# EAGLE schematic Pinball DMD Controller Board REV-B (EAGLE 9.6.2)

## Sheet 1 of 6: Clock / Sync
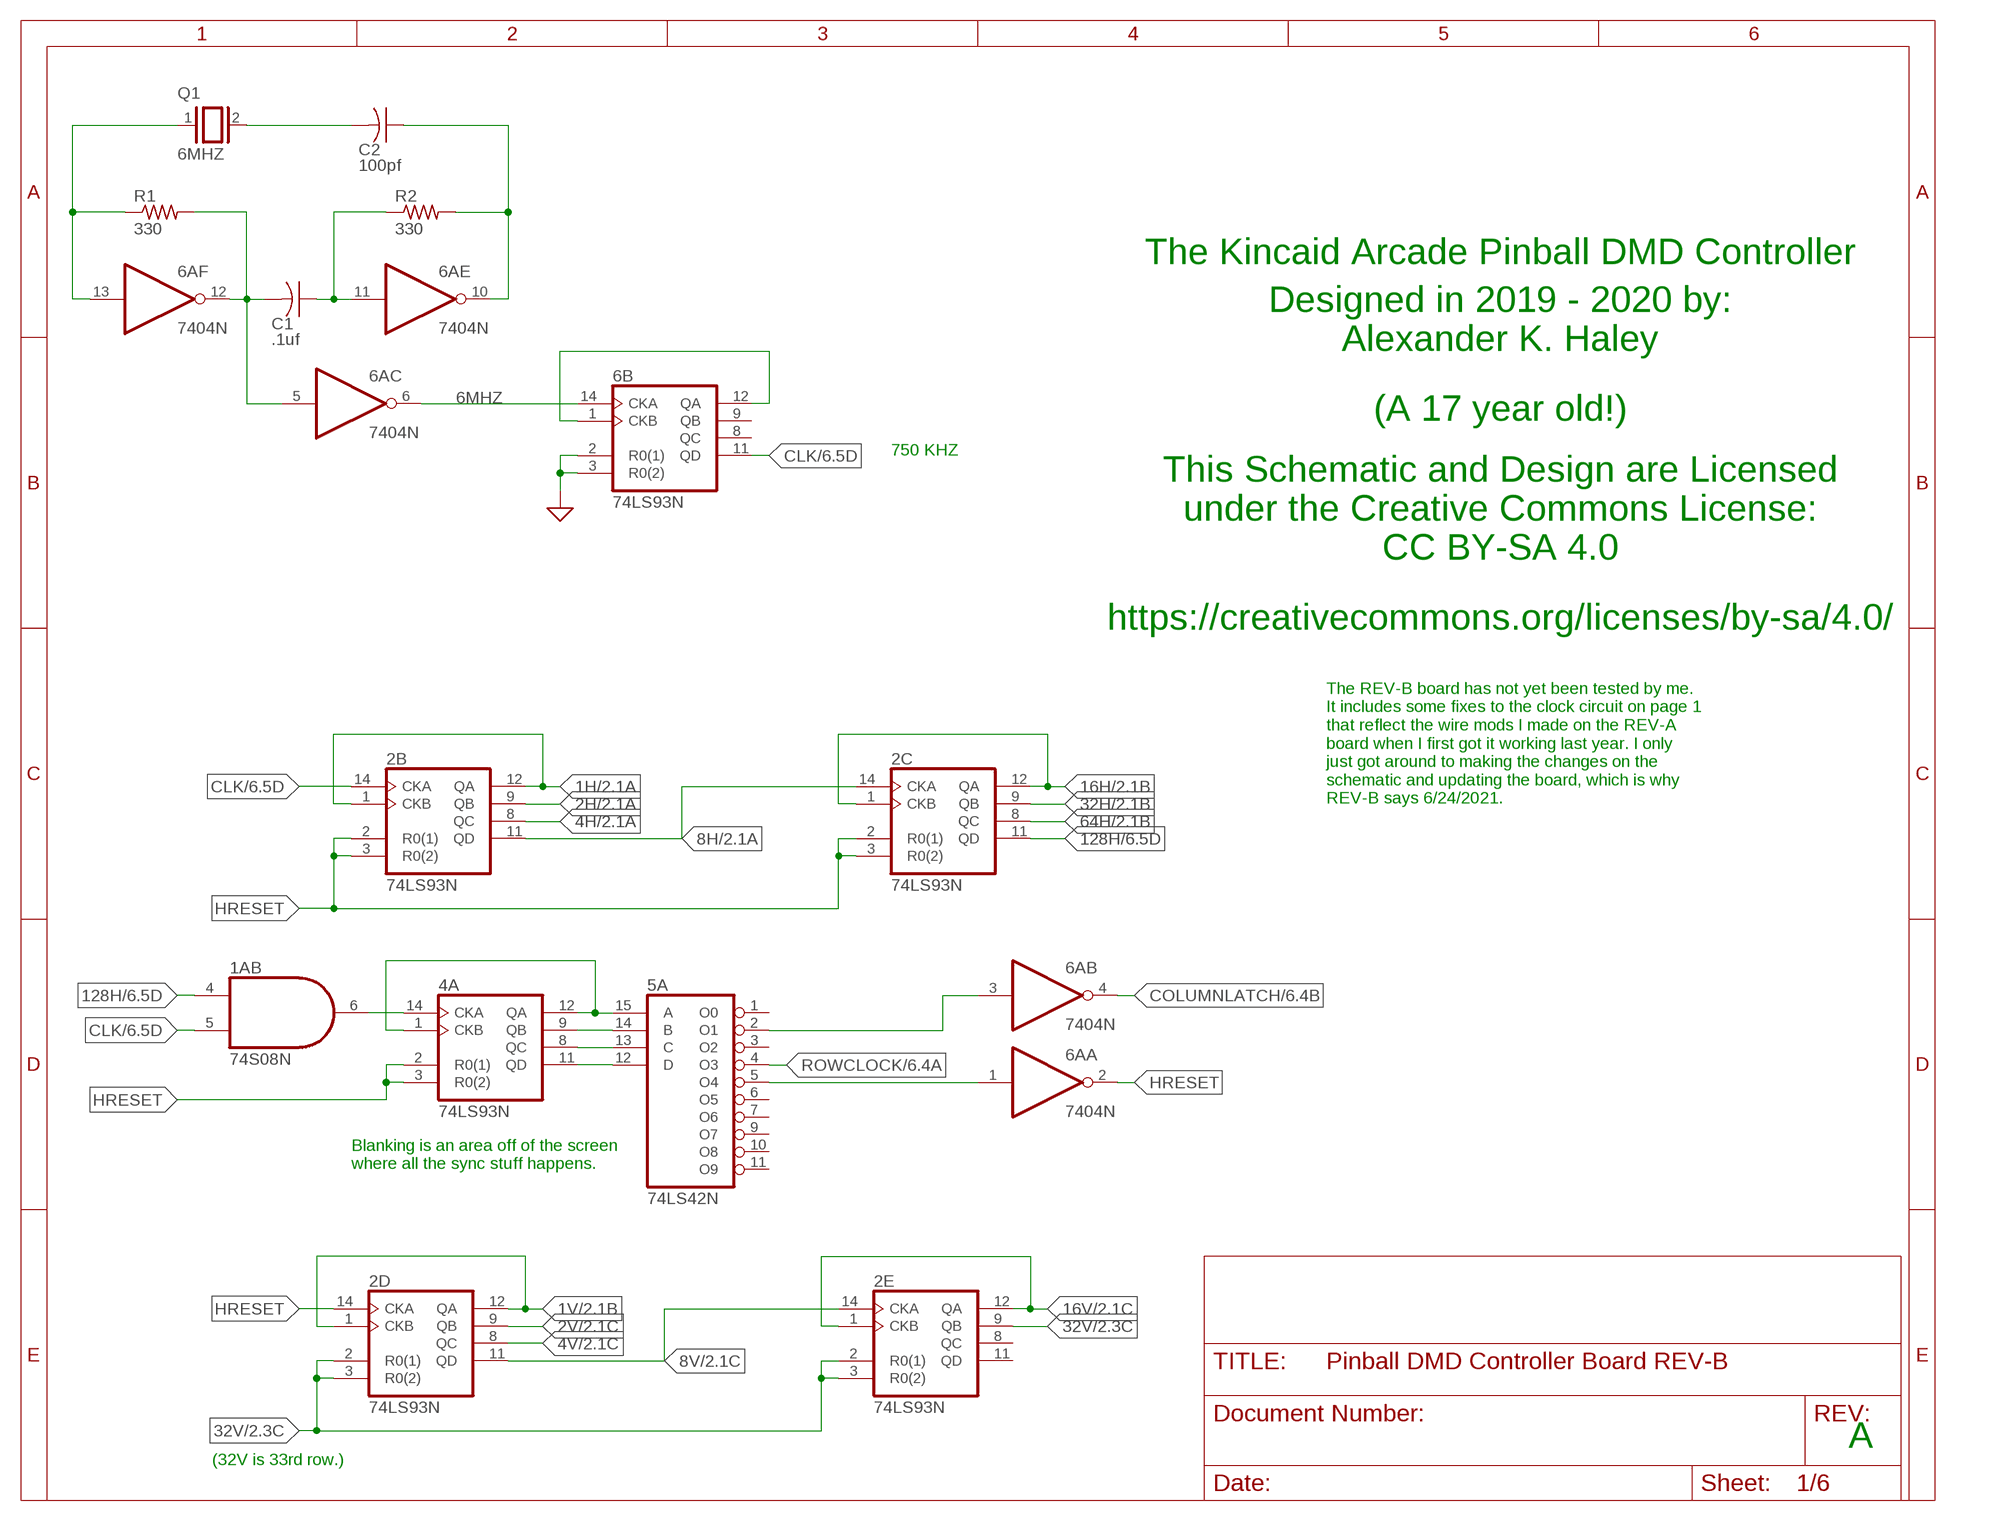
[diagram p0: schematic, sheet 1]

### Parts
1A  74S08N  [DIL14]
2B  74LS93N  [DIL14]
2C  74LS93N  [DIL14]
2D  74LS93N  [DIL14]
2E  74LS93N  [DIL14]
4A  74LS93N  [DIL14]
5A  74LS42N  [DIL16]
6A  7404N  [DIL14]
6B  74LS93N  [DIL14]
C1  .1uf  C-US050-025X075  [C050-025X075]
C2  100pf  C-US050-025X075  [C050-025X075]
Q1  6MHZ  XTAL/S  [QS]
R1  330  R-US_0204/7  [0204/7]
R2  330  R-US_0204/7  [0204/7]

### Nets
1H: 2B.1(CKB) 2B.12(QA) ; also sheet 2,3
1V: 2D.1(CKB) 2D.12(QA) ; also sheet 2,3,6
2H: 2B.9(QB) ; also sheet 2,3
2V: 2D.9(QB) ; also sheet 2,3,6
4H: 2B.8(QC) ; also sheet 2,3
4V: 2D.8(QC) ; also sheet 2,3,6
6MHZ: 6A.6(C:O) 6B.14(CKA) ; also sheet 4
8H: 2B.11(QD) 2C.14(CKA) ; also sheet 2,3
8V: 2D.11(QD) 2E.14(CKA) ; also sheet 2,3,6
16H: 2C.1(CKB) 2C.12(QA) ; also sheet 2,3
16V: 2E.1(CKB) 2E.12(QA) ; also sheet 2,3,6
32H: 2C.9(QB) ; also sheet 2,3
32V: 2D.2(R0(1)) 2D.3(R0(2)) 2E.2(R0(1)) 2E.3(R0(2)) 2E.9(QB) ; also sheet 2
64H: 2C.8(QC) ; also sheet 2,3
128H: 1A.4(B:I0) 2C.11(QD) ; also sheet 6
CLK: 1A.5(B:I1) 2B.14(CKA) 6B.11(QD) ; also sheet 6
COLUMNLATCH: 6A.4(B:O) ; also sheet 6
GND: 6B.2(R0(1)) 6B.3(R0(2)) ; supply symbol labelled SUP ; also sheet 2,3,4,5,6
HRESET: 2B.2(R0(1)) 2B.3(R0(2)) 2C.2(R0(1)) 2C.3(R0(2)) 2D.14(CKA) 4A.2(R0(1)) 4A.3(R0(2)) 6A.2(A:O)
N$1: 6A.13(F:I) Q1.1 R1.1
N$2: 6A.5(C:I) 6A.12(F:O) C1.2 R1.2
N$3: 6A.11(E:I) C1.1 R2.1
N$4: C2.2 Q1.2
N$5: 6A.10(E:O) C2.1 R2.2
N$7: 6B.1(CKB) 6B.12(QA)
N$14: 1A.6(B:O) 4A.14(CKA)
N$15: 4A.1(CKB) 4A.12(QA) 5A.15(A)
N$17: 4A.9(QB) 5A.14(B)
N$18: 4A.8(QC) 5A.13(C)
N$19: 4A.11(QD) 5A.12(D)
N$20: 5A.5(O4) 6A.1(A:I)
N$21: 5A.2(O1) 6A.3(B:I)
ROWCLOCK: 5A.4(O3) ; also sheet 6
Unconnected: 2E.8(QC) 2E.11(QD) 5A.1(O0) 5A.3(O2) 5A.6(O5) 5A.7(O6) 5A.9(O7) 5A.10(O8) 5A.11(O9) 6B.8(QC) 6B.9(QB)

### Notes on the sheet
- The Kincaid Arcade Pinball DMD Controller
- Designed in 2019 - 2020 by:
  Alexander K. Haley
- (A 17 year old!)
- 750 KHZ
- This Schematic and Design are Licensed
  under the Creative Commons License:
  CC BY-SA 4.0
- https://creativecommons.org/licenses/by-sa/4.0/
- The REV-B board has not yet been tested by me.
  It includes some fixes to the clock circuit on page 1
  that reflect the wire mods I made on the REV-A
  board when I first got it working last year. I only
  just got around to making the changes on the
  schematic and updating the board, which is why
  REV-B says 6/24/2021.
- Blanking is an area off of the screen
  where all the sync stuff happens.
- A
- (32V is 33rd row.)

## Sheet 2 of 6: Memory A
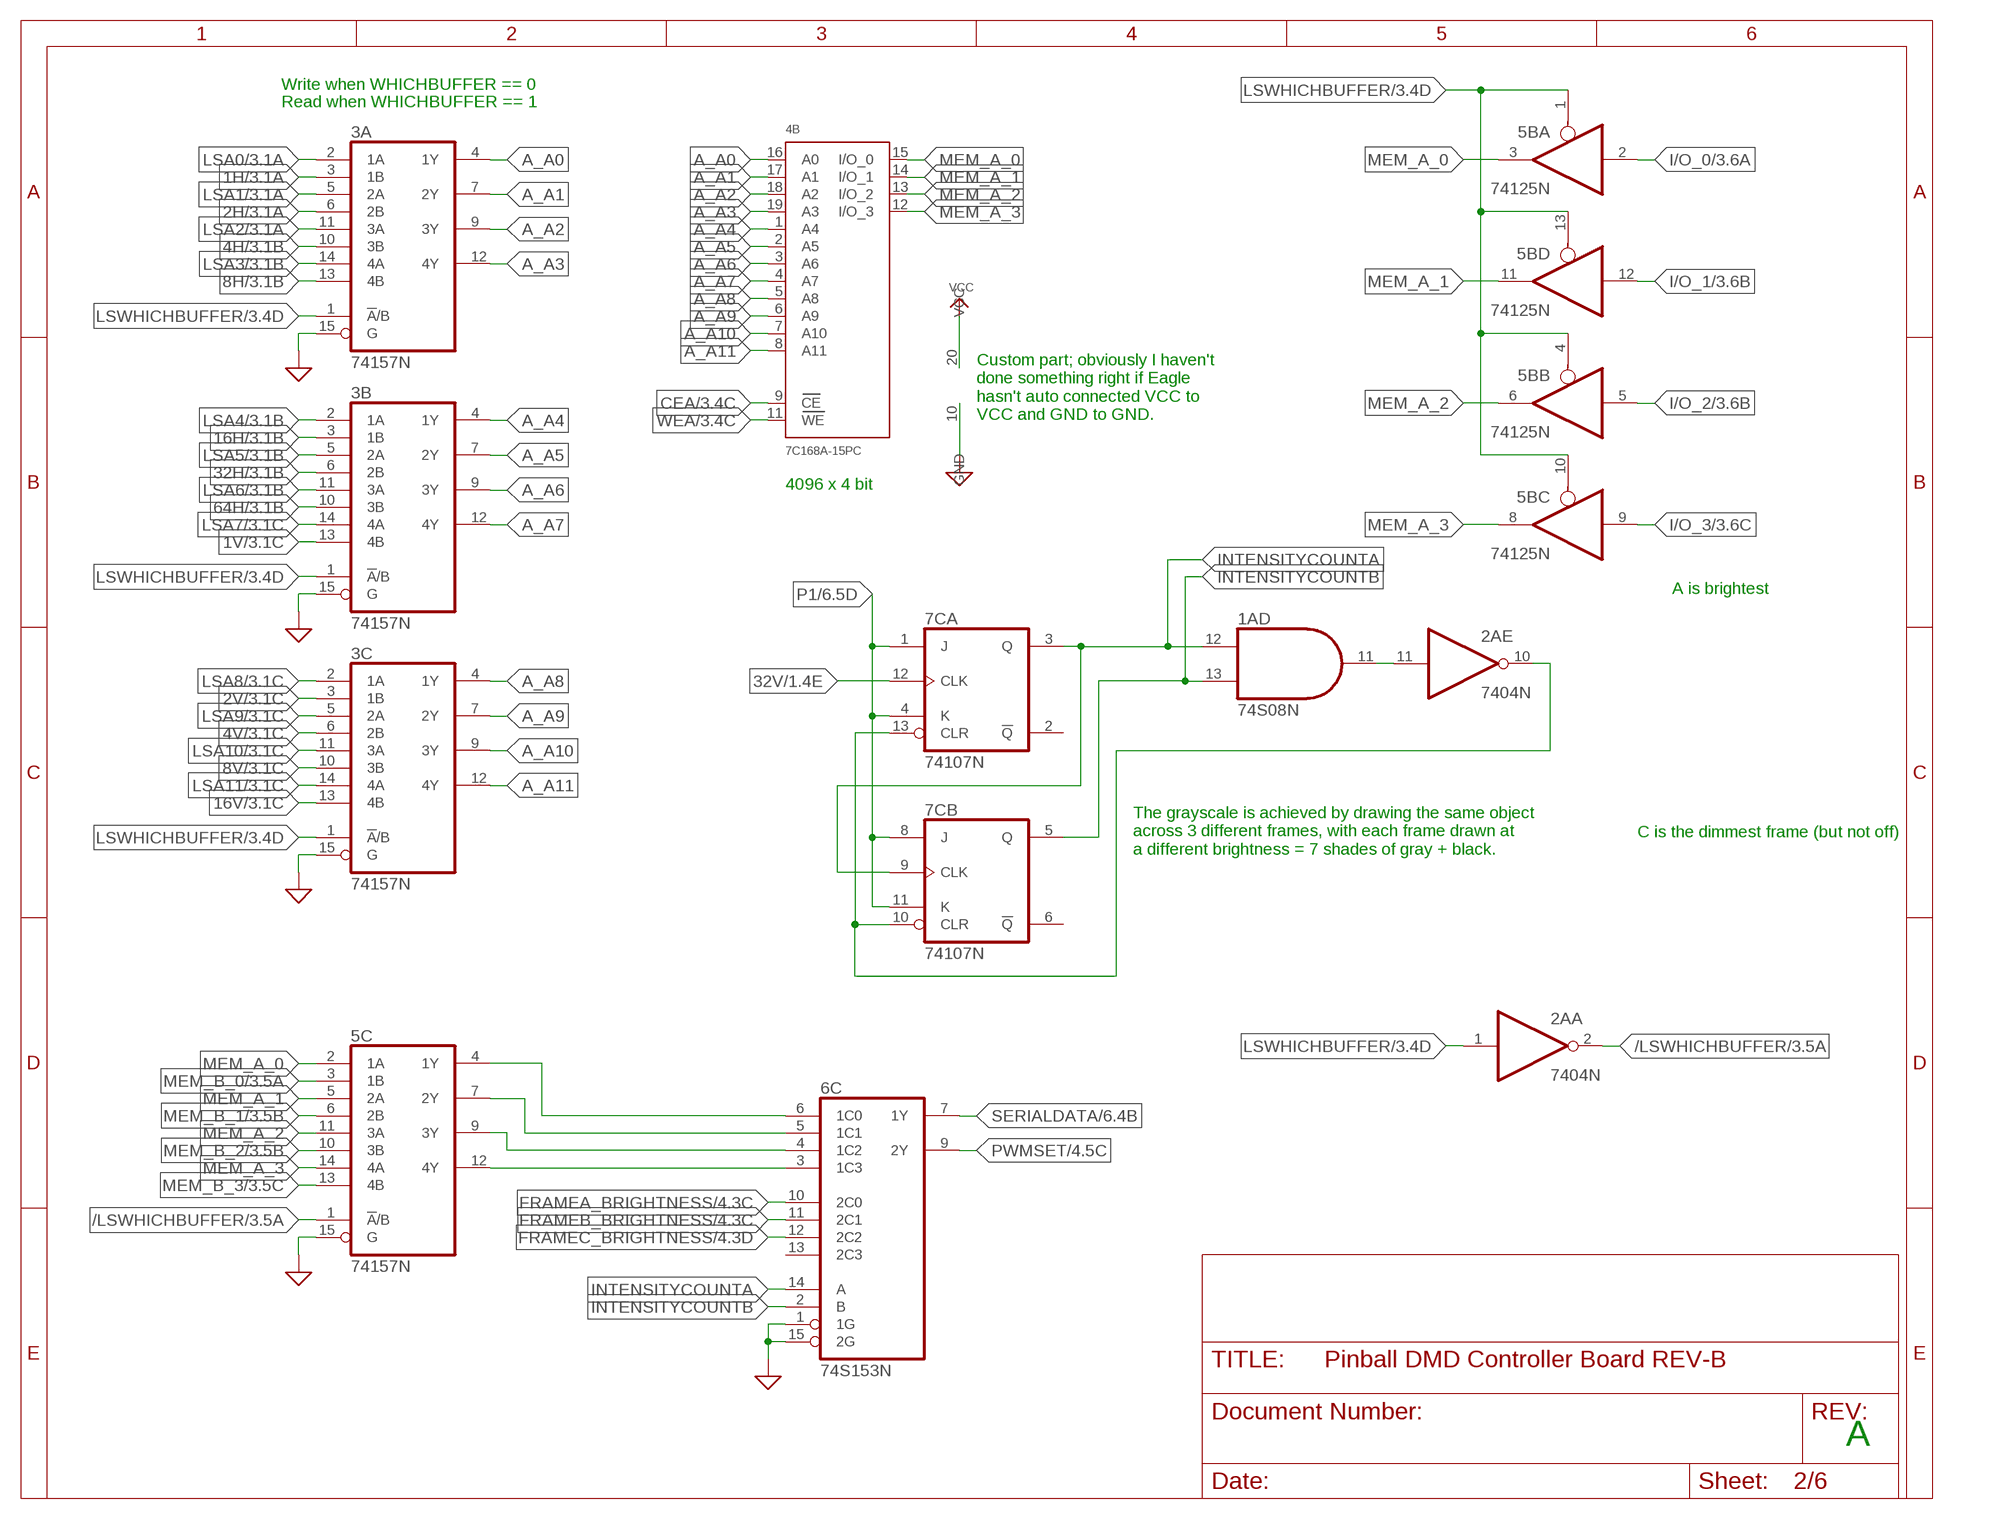
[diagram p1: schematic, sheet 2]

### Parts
2A  7404N  [DIL14]
3A  74157N  [DIL16]
3B  74157N  [DIL16]
3C  74157N  [DIL16]
4B  7C168A-15PC  [DIL20]
5B  74125N  [DIL14]
5C  74157N  [DIL16]
6C  74S153N  [DIL16]
7C  74107N  [DIL14]

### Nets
1H: 3A.3(1B) ; also sheet 1,3
1V: 3B.13(4B) ; also sheet 1,3,6
2H: 3A.6(2B) ; also sheet 1,3
2V: 3C.3(1B) ; also sheet 1,3,6
4H: 3A.10(3B) ; also sheet 1,3
4V: 3C.6(2B) ; also sheet 1,3,6
8H: 3A.13(4B) ; also sheet 1,3
8V: 3C.10(3B) ; also sheet 1,3,6
16H: 3B.3(1B) ; also sheet 1,3
16V: 3C.13(4B) ; also sheet 1,3,6
32H: 3B.6(2B) ; also sheet 1,3
32V: 7C.12(A:CLK) ; also sheet 1
64H: 3B.10(3B) ; also sheet 1,3
/LSWHICHBUFFER: 2A.2(A:O) 5C.1(!A!/B) ; also sheet 3
A_A0: 3A.4(1Y) 4B.16(A0)
A_A1: 3A.7(2Y) 4B.17(A1)
A_A2: 3A.9(3Y) 4B.18(A2)
A_A3: 3A.12(4Y) 4B.19(A3)
A_A4: 3B.4(1Y) 4B.1(A4)
A_A5: 3B.7(2Y) 4B.2(A5)
A_A6: 3B.9(3Y) 4B.3(A6)
A_A7: 3B.12(4Y) 4B.4(A7)
A_A8: 3C.4(1Y) 4B.5(A8)
A_A9: 3C.7(2Y) 4B.6(A9)
A_A10: 3C.9(3Y) 4B.7(A10)
A_A11: 3C.12(4Y) 4B.8(A11)
CEA: 4B.9(CE) ; also sheet 3
FRAMEA_BRIGHTNESS: 6C.10(2C0) ; also sheet 4
FRAMEB_BRIGHTNESS: 6C.11(2C1) ; also sheet 4
FRAMEC_BRIGHTNESS: 6C.12(2C2) ; also sheet 4
GND: 3A.15(G) 3B.15(G) 3C.15(G) 4B.10(GND) 5C.15(G) 6C.1(1G) 6C.15(2G) ; supply symbol labelled SUP ; also sheet 1,3,4,5,6
I/O_0: 5B.2(A:I) ; also sheet 3,5
I/O_1: 5B.12(D:I) ; also sheet 3,5
I/O_2: 5B.5(B:I) ; also sheet 3,5
I/O_3: 5B.9(C:I) ; also sheet 3,5
INTENSITYCOUNTA: 1A.12(D:I0) 6C.14(A) 7C.3(A:Q) 7C.9(B:CLK)
INTENSITYCOUNTB: 1A.13(D:I1) 6C.2(B) 7C.5(B:Q)
LSA0: 3A.2(1A) ; also sheet 3,5
LSA1: 3A.5(2A) ; also sheet 3,5
LSA2: 3A.11(3A) ; also sheet 3,5
LSA3: 3A.14(4A) ; also sheet 3,5
LSA4: 3B.2(1A) ; also sheet 3,5
LSA5: 3B.5(2A) ; also sheet 3,5
LSA6: 3B.11(3A) ; also sheet 3,5
LSA7: 3B.14(4A) ; also sheet 3,5
LSA8: 3C.2(1A) ; also sheet 3,5
LSA9: 3C.5(2A) ; also sheet 3,5
LSA10: 3C.11(3A) ; also sheet 3,5
LSA11: 3C.14(4A) ; also sheet 3,5
LSWHICHBUFFER: 2A.1(A:I) 3A.1(!A!/B) 3B.1(!A!/B) 3C.1(!A!/B) 5B.1(A:OE) 5B.4(B:OE) 5B.10(C:OE) 5B.13(D:OE) ; also sheet 3,5
MEM_A_0: 4B.15(I/O_0) 5B.3(A:O) 5C.2(1A)
MEM_A_1: 4B.14(I/O_1) 5B.11(D:O) 5C.5(2A)
MEM_A_2: 4B.13(I/O_2) 5B.6(B:O) 5C.11(3A)
MEM_A_3: 4B.12(I/O_3) 5B.8(C:O) 5C.14(4A)
MEM_B_0: 5C.3(1B) ; also sheet 3
MEM_B_1: 5C.6(2B) ; also sheet 3
MEM_B_2: 5C.10(3B) ; also sheet 3
MEM_B_3: 5C.13(4B) ; also sheet 3
N$6: 1A.11(D:O) 2A.11(E:I)
N$23: 2A.10(E:O) 7C.10(B:CLR) 7C.13(A:CLR)
N$25: 5C.12(4Y) 6C.3(1C3)
N$26: 5C.9(3Y) 6C.4(1C2)
N$36: 5C.7(2Y) 6C.5(1C1)
N$39: 5C.4(1Y) 6C.6(1C0)
P1: 7C.1(A:J) 7C.4(A:K) 7C.8(B:J) 7C.11(B:K) ; also sheet 6
PWMSET: 6C.9(2Y) ; also sheet 4
SERIALDATA: 6C.7(1Y) ; also sheet 6
VCC: 4B.20(VCC) ; also sheet 3,5,6
WEA: 4B.11(WE) ; also sheet 3
Unconnected: 6C.13(2C3) 7C.2(A:!Q) 7C.6(B:!Q)

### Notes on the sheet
- Write when WHICHBUFFER == 0
- Read when WHICHBUFFER == 1
- Custom part; obviously I haven't
  done something right if Eagle 
  hasn't auto connected VCC to
  VCC and GND to GND.
- 4096 x 4 bit
- A is brightest
- C is the dimmest frame (but not off)
- The grayscale is achieved by drawing the same object
  across 3 different frames, with each frame drawn at 
  a different brightness = 7 shades of gray + black.
- A

## Sheet 3 of 6: Memory B
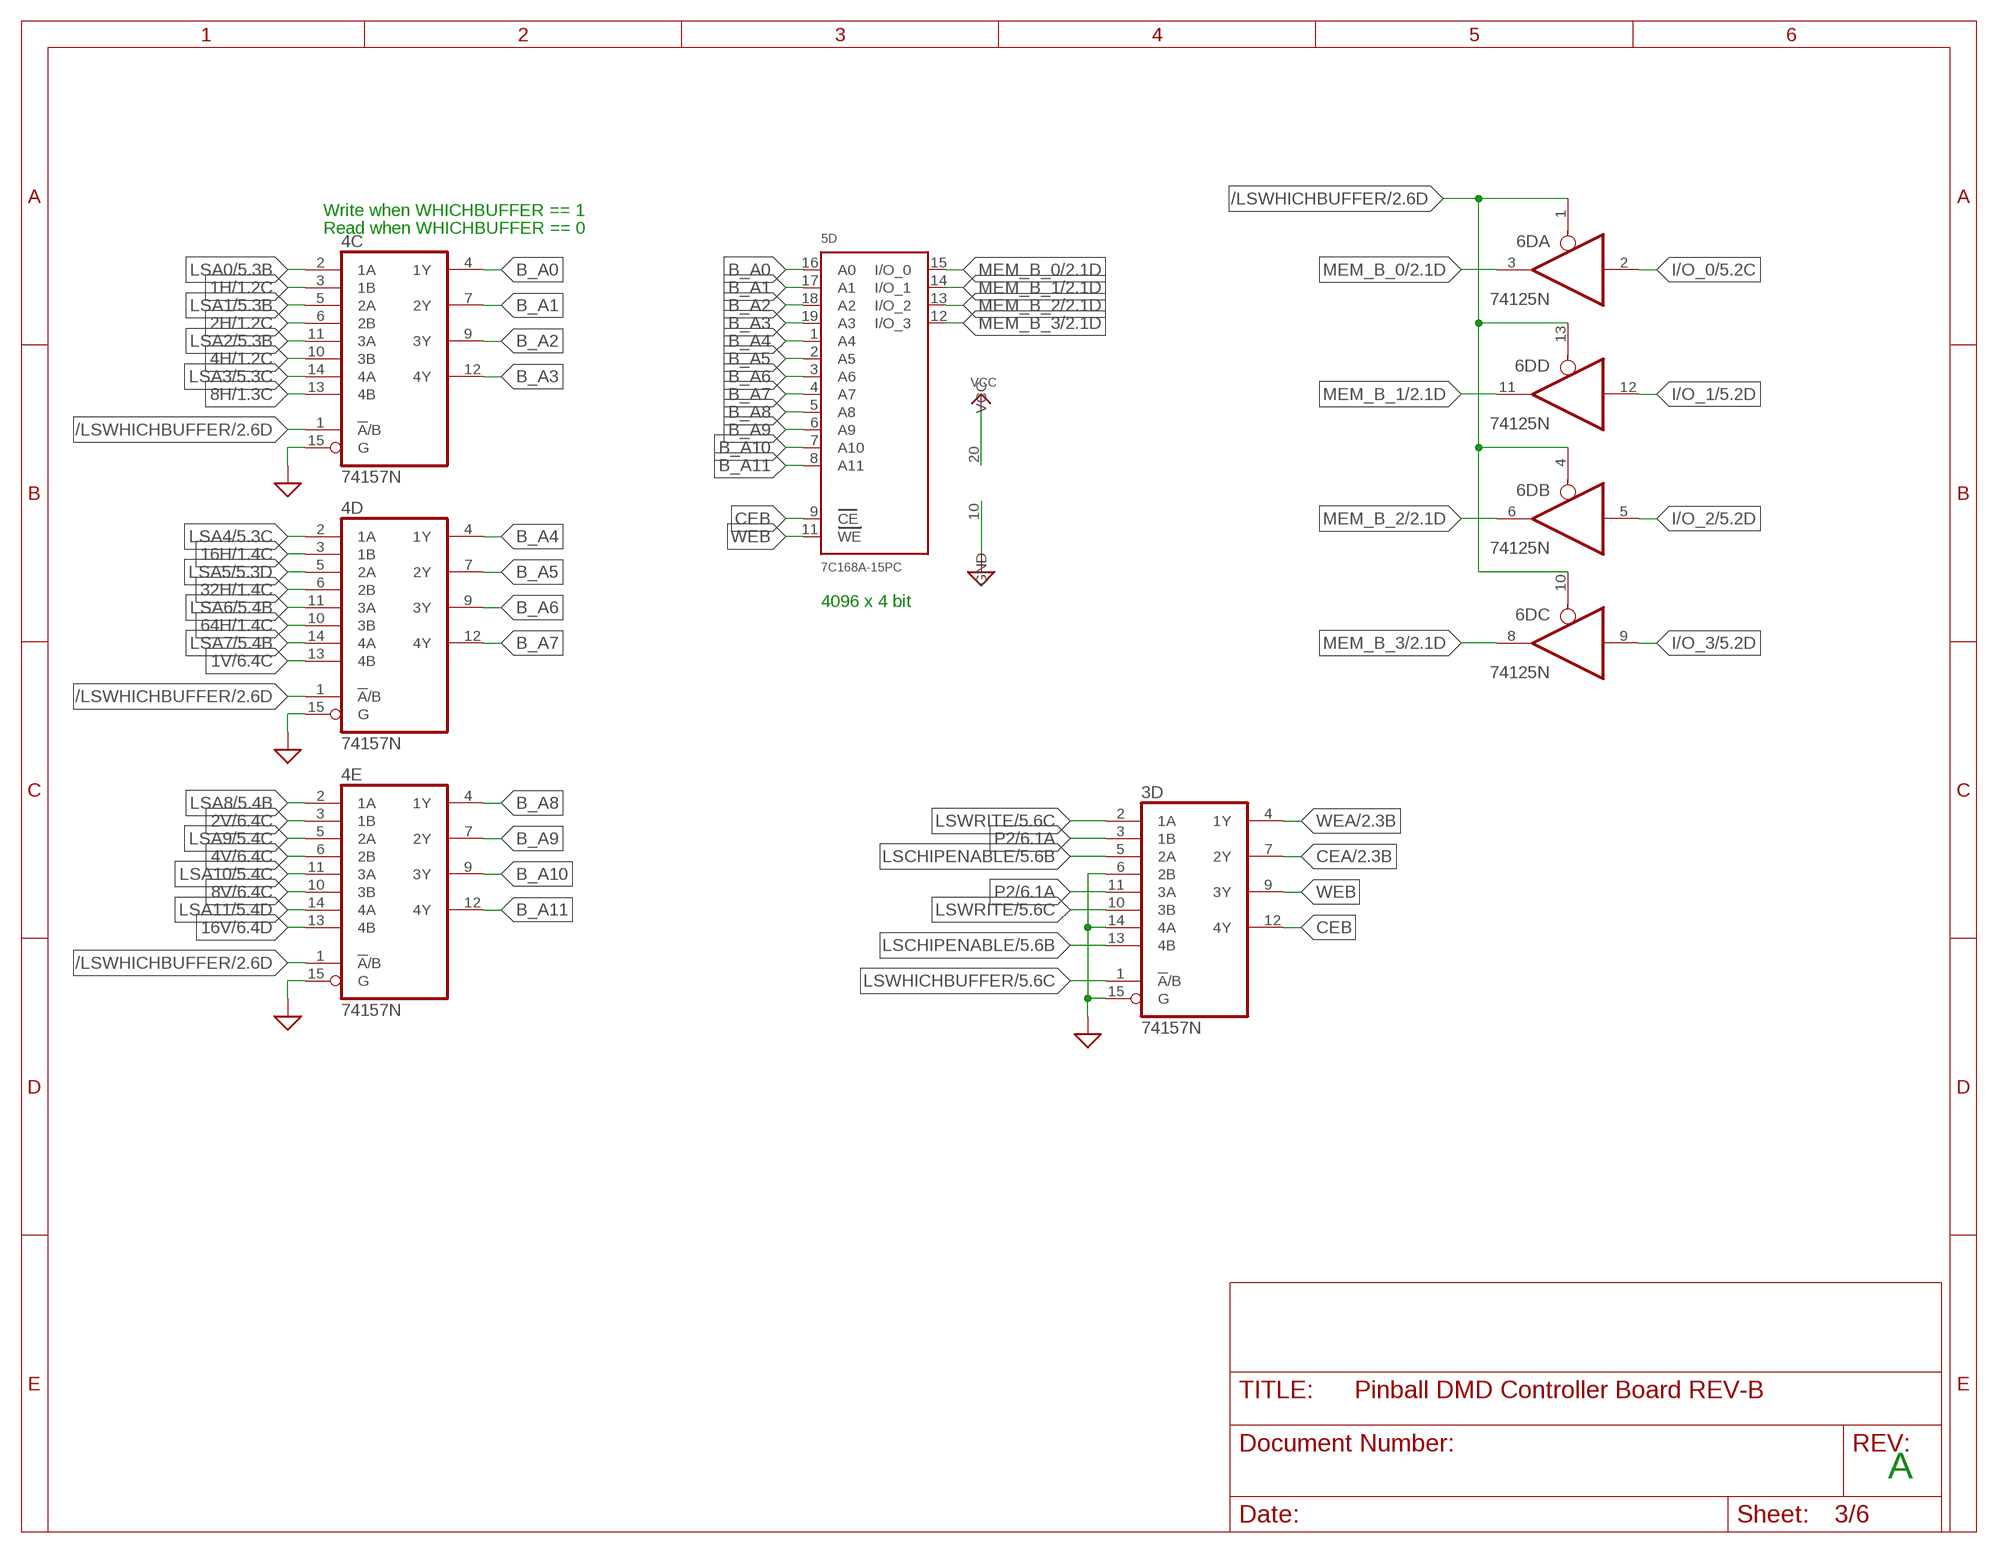
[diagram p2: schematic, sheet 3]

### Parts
3D  74157N  [DIL16]
4C  74157N  [DIL16]
4D  74157N  [DIL16]
4E  74157N  [DIL16]
5D  7C168A-15PC  [DIL20]
6D  74125N  [DIL14]

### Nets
1H: 4C.3(1B) ; also sheet 1,2
1V: 4D.13(4B) ; also sheet 1,2,6
2H: 4C.6(2B) ; also sheet 1,2
2V: 4E.3(1B) ; also sheet 1,2,6
4H: 4C.10(3B) ; also sheet 1,2
4V: 4E.6(2B) ; also sheet 1,2,6
8H: 4C.13(4B) ; also sheet 1,2
8V: 4E.10(3B) ; also sheet 1,2,6
16H: 4D.3(1B) ; also sheet 1,2
16V: 4E.13(4B) ; also sheet 1,2,6
32H: 4D.6(2B) ; also sheet 1,2
64H: 4D.10(3B) ; also sheet 1,2
/LSWHICHBUFFER: 4C.1(!A!/B) 4D.1(!A!/B) 4E.1(!A!/B) 6D.1(A:OE) 6D.4(B:OE) 6D.10(C:OE) 6D.13(D:OE) ; also sheet 2
B_A0: 4C.4(1Y) 5D.16(A0)
B_A1: 4C.7(2Y) 5D.17(A1)
B_A2: 4C.9(3Y) 5D.18(A2)
B_A3: 4C.12(4Y) 5D.19(A3)
B_A4: 4D.4(1Y) 5D.1(A4)
B_A5: 4D.7(2Y) 5D.2(A5)
B_A6: 4D.9(3Y) 5D.3(A6)
B_A7: 4D.12(4Y) 5D.4(A7)
B_A8: 4E.4(1Y) 5D.5(A8)
B_A9: 4E.7(2Y) 5D.6(A9)
B_A10: 4E.9(3Y) 5D.7(A10)
B_A11: 4E.12(4Y) 5D.8(A11)
CEA: 3D.7(2Y) ; also sheet 2
CEB: 3D.12(4Y) 5D.9(CE)
GND: 3D.6(2B) 3D.14(4A) 3D.15(G) 4C.15(G) 4D.15(G) 4E.15(G) 5D.10(GND) ; supply symbol labelled SUP ; also sheet 1,2,4,5,6
I/O_0: 6D.2(A:I) ; also sheet 2,5
I/O_1: 6D.12(D:I) ; also sheet 2,5
I/O_2: 6D.5(B:I) ; also sheet 2,5
I/O_3: 6D.9(C:I) ; also sheet 2,5
LSA0: 4C.2(1A) ; also sheet 2,5
LSA1: 4C.5(2A) ; also sheet 2,5
LSA2: 4C.11(3A) ; also sheet 2,5
LSA3: 4C.14(4A) ; also sheet 2,5
LSA4: 4D.2(1A) ; also sheet 2,5
LSA5: 4D.5(2A) ; also sheet 2,5
LSA6: 4D.11(3A) ; also sheet 2,5
LSA7: 4D.14(4A) ; also sheet 2,5
LSA8: 4E.2(1A) ; also sheet 2,5
LSA9: 4E.5(2A) ; also sheet 2,5
LSA10: 4E.11(3A) ; also sheet 2,5
LSA11: 4E.14(4A) ; also sheet 2,5
LSCHIPENABLE: 3D.5(2A) 3D.13(4B) ; also sheet 5
LSWHICHBUFFER: 3D.1(!A!/B) ; also sheet 2,5
LSWRITE: 3D.2(1A) 3D.10(3B) ; also sheet 5
MEM_B_0: 5D.15(I/O_0) 6D.3(A:O) ; also sheet 2
MEM_B_1: 5D.14(I/O_1) 6D.11(D:O) ; also sheet 2
MEM_B_2: 5D.13(I/O_2) 6D.6(B:O) ; also sheet 2
MEM_B_3: 5D.12(I/O_3) 6D.8(C:O) ; also sheet 2
P2: 3D.3(1B) 3D.11(3A) ; also sheet 6
VCC: 5D.20(VCC) ; also sheet 2,5,6
WEA: 3D.4(1Y) ; also sheet 2
WEB: 3D.9(3Y) 5D.11(WE)

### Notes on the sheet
- Write when WHICHBUFFER == 1
- Read when WHICHBUFFER == 0
- 4096 x 4 bit
- A

## Sheet 4 of 6: PWM
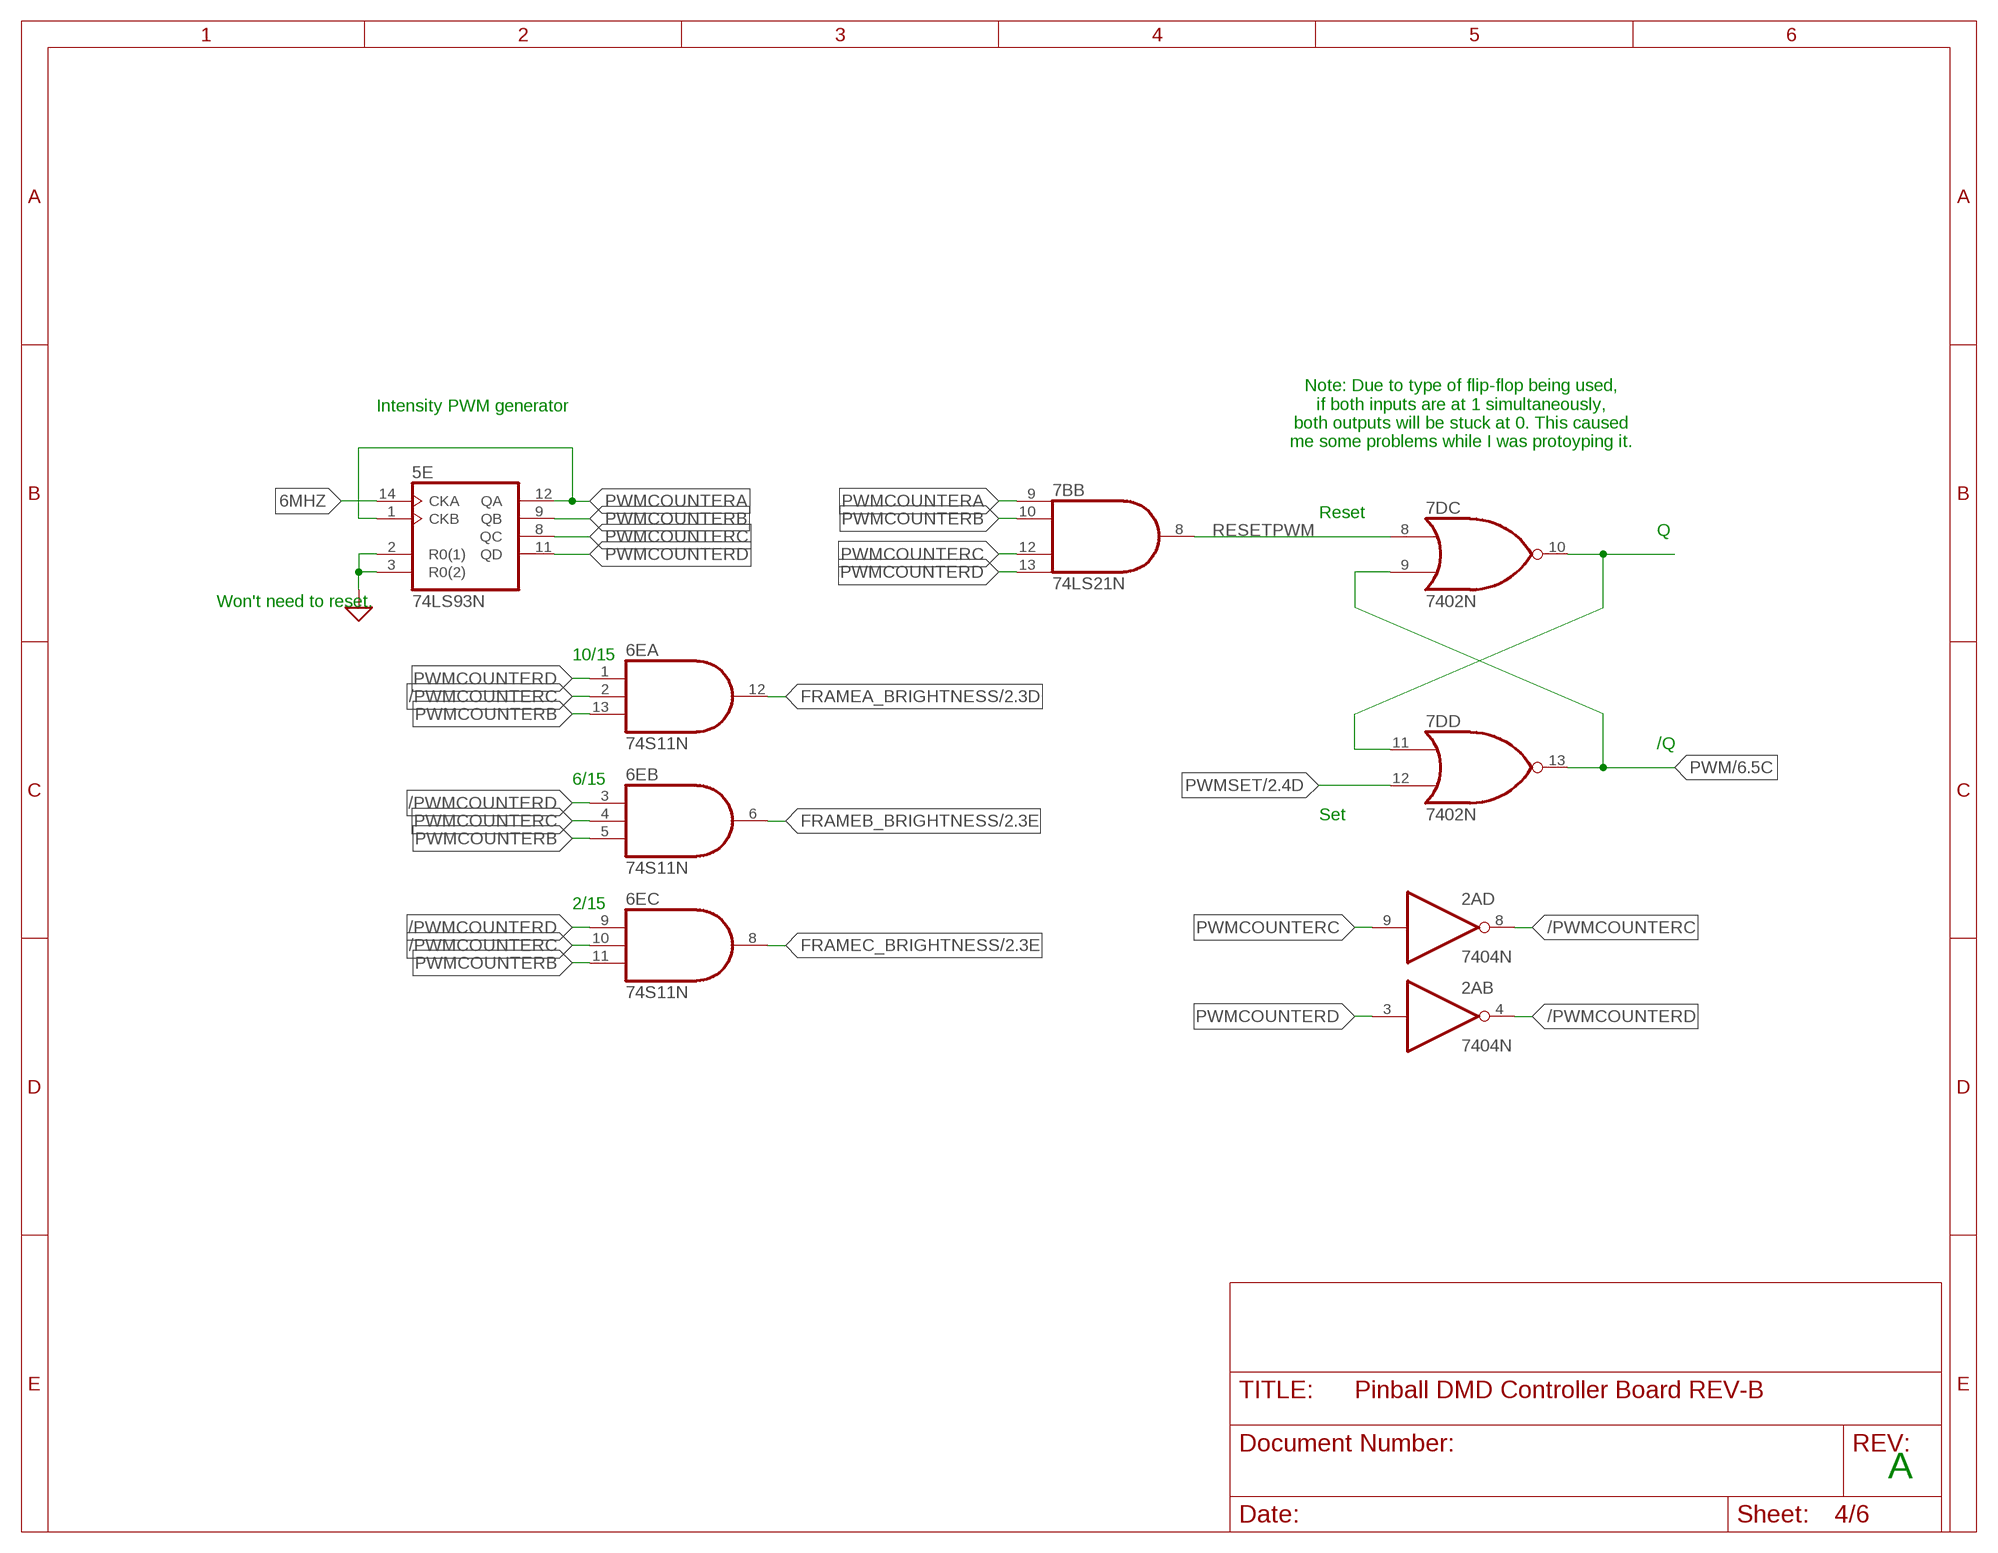
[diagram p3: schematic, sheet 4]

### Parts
5E  74LS93N  [DIL14]
6E  74S11N  [DIL14]
7B  74LS21N  [DIL14]
7D  7402N  [DIL14]

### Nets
6MHZ: 5E.14(CKA) ; also sheet 1
/PWMCOUNTERC: 2A.8(D:O) 6E.2(A:I1) 6E.10(C:I1)
/PWMCOUNTERD: 2A.4(B:O) 6E.3(B:I0) 6E.9(C:I0)
FRAMEA_BRIGHTNESS: 6E.12(A:O) ; also sheet 2
FRAMEB_BRIGHTNESS: 6E.6(B:O) ; also sheet 2
FRAMEC_BRIGHTNESS: 6E.8(C:O) ; also sheet 2
GND: 5E.2(R0(1)) 5E.3(R0(2)) ; supply symbol labelled SUP ; also sheet 1,2,3,5,6
N$22: 7D.10(C:O) 7D.11(D:I0)
PWM: 7D.9(C:I1) 7D.13(D:O) ; also sheet 6
PWMCOUNTERA: 5E.1(CKB) 5E.12(QA) 7B.9(B:I0)
PWMCOUNTERB: 5E.9(QB) 6E.5(B:I2) 6E.11(C:I2) 6E.13(A:I2) 7B.10(B:I1)
PWMCOUNTERC: 2A.9(D:I) 5E.8(QC) 6E.4(B:I1) 7B.12(B:I2)
PWMCOUNTERD: 2A.3(B:I) 5E.11(QD) 6E.1(A:I0) 7B.13(B:I3)
PWMSET: 7D.12(D:I1) ; also sheet 2
RESETPWM: 7B.8(B:O) 7D.8(C:I0)

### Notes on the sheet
- Intensity PWM generator
- Note: Due to type of flip-flop being used,
  if both inputs are at 1 simultaneously,
  both outputs will be stuck at 0. This caused
  me some problems while I was protoyping it.
- Reset
- Q
- Won't need to reset.
- 10/15
- /Q
- 6/15
- Set
- 2/15
- A

## Sheet 5 of 6: Level Shifting
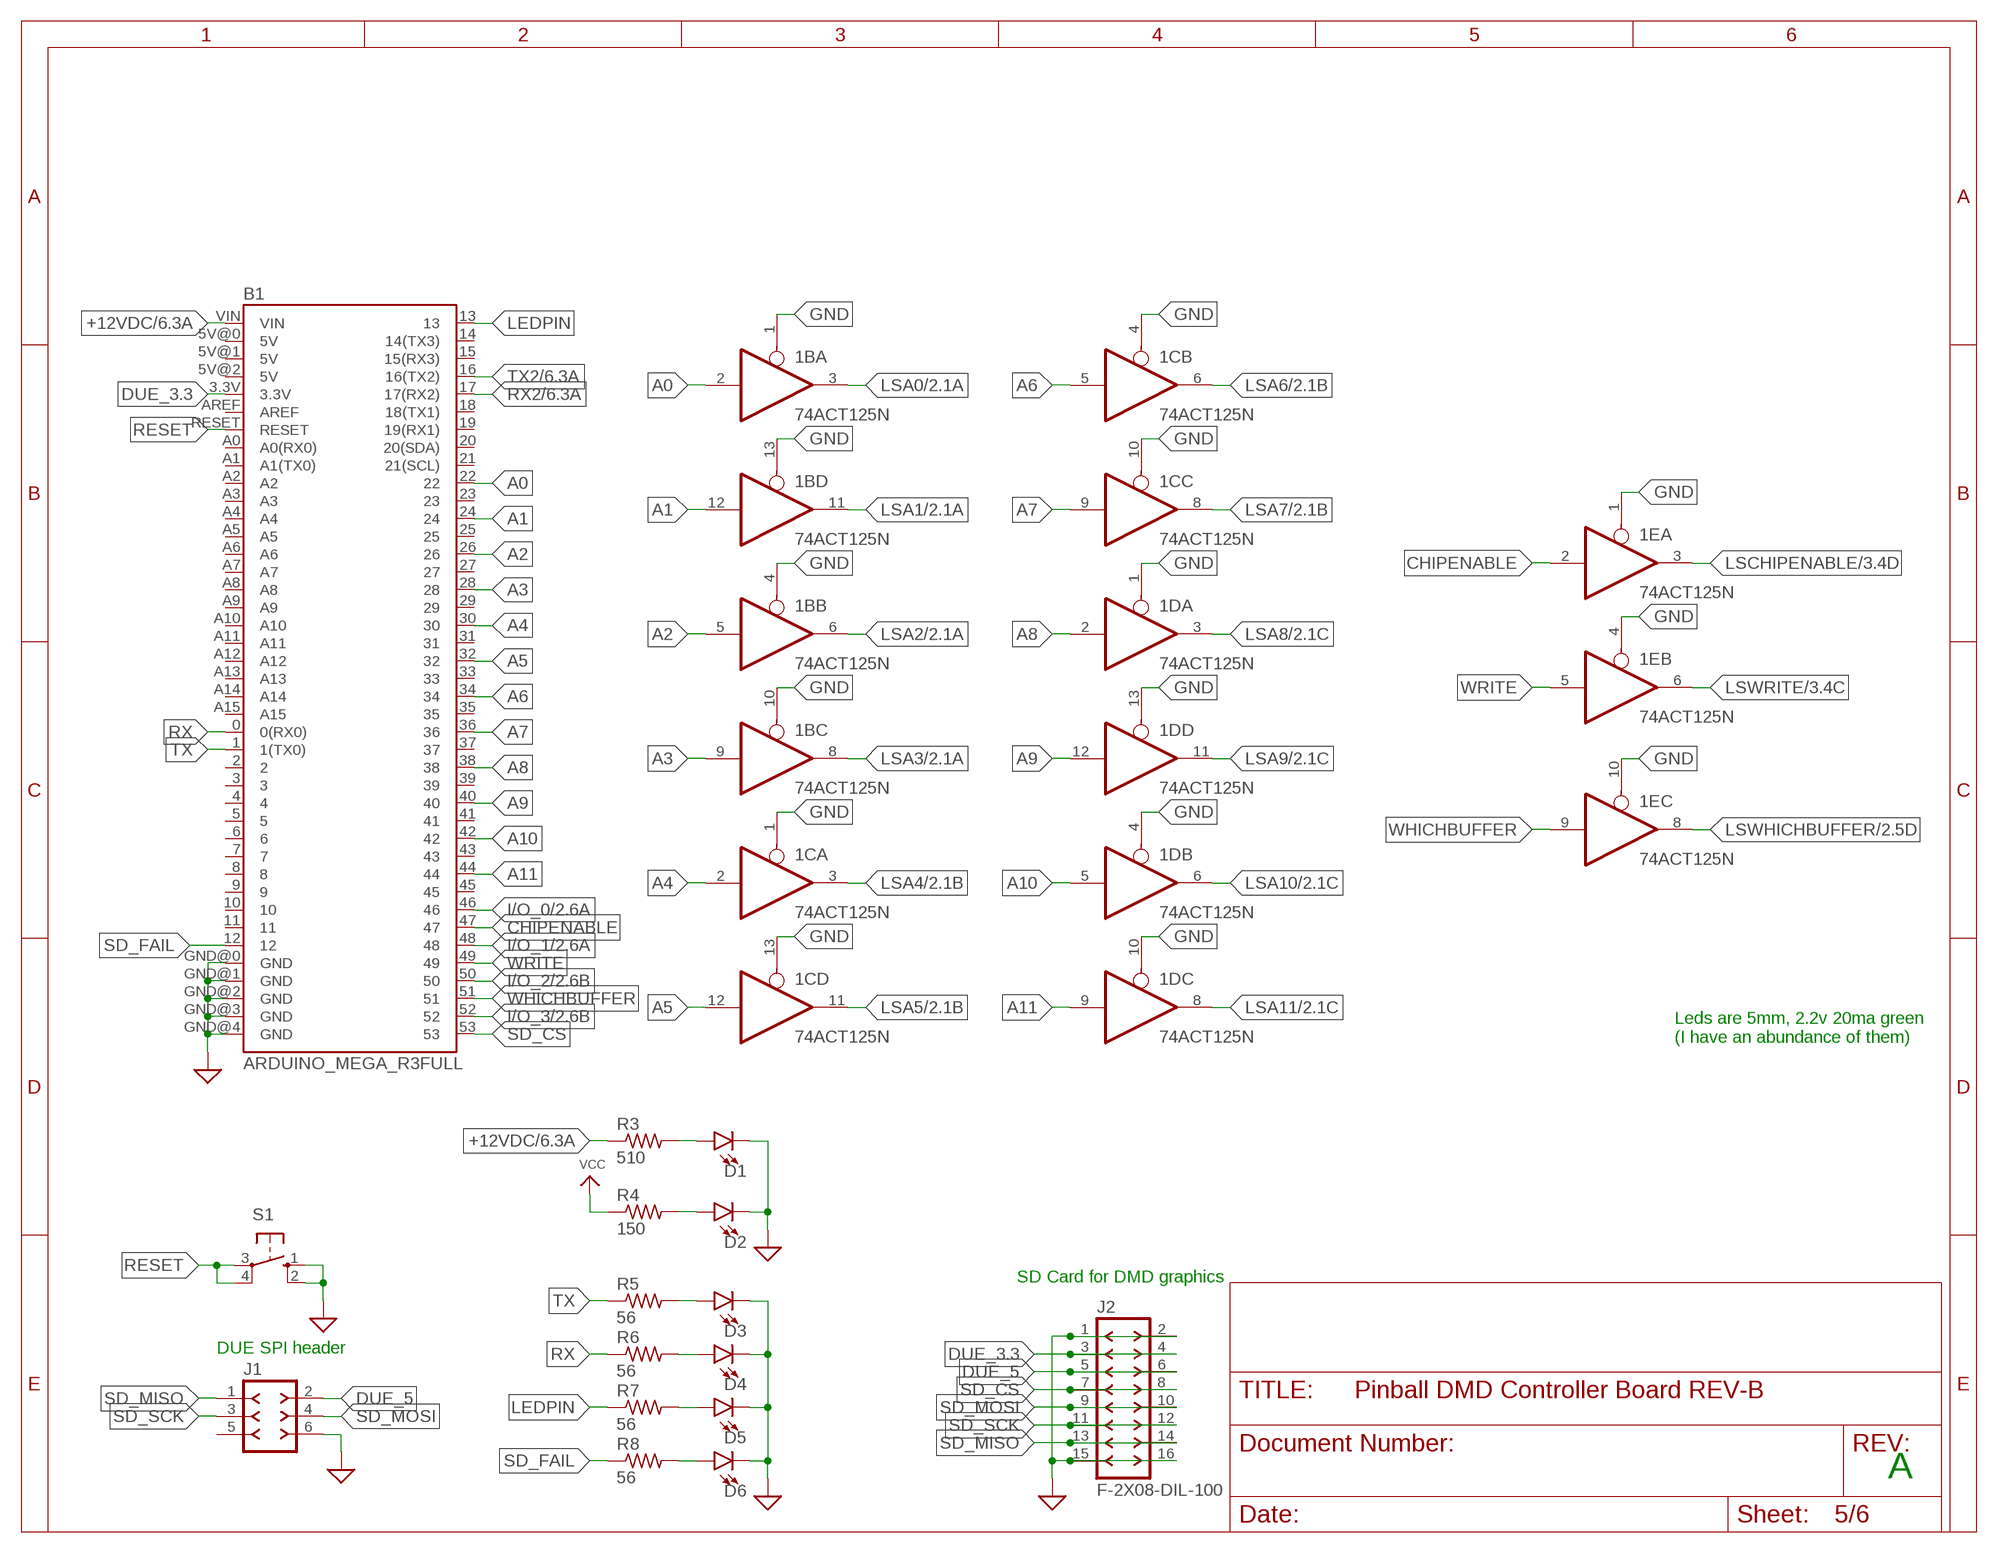
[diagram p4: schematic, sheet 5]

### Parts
1B  74ACT125N  74125N  [DIL14]
1C  74ACT125N  74125N  [DIL14]
1D  74ACT125N  74125N  [DIL14]
1E  74ACT125N  74125N  [DIL14]
B1  ARDUINO_MEGA_R3FULL  [ARDUINO_MEGA]
D1  LED5MM  [LED_5MM]
D2  LED5MM  [LED_5MM]
D3  LED5MM  [LED_5MM]
D4  LED5MM  [LED_5MM]
D5  LED5MM  [LED_5MM]
D6  LED5MM  [LED_5MM]
J1  F-2X03-DIL-100  [DIL-100-2X03]
J2  F-2X08-DIL-100  [DIL-100-2X08]
R3  510  R-US_0204/7  [0204/7]
R4  150  R-US_0204/7  [0204/7]
R5  56  R-US_0204/7  [0204/7]
R6  56  R-US_0204/7  [0204/7]
R7  56  R-US_0204/7  [0204/7]
R8  56  R-US_0204/7  [0204/7]
S1  10-XX  [B3F-10XX]

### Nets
+12VDC: B1.VIN R3.1 ; also sheet 6
A0: 1B.2(A:I) B1.22
A1: 1B.12(D:I) B1.24
A2: 1B.5(B:I) B1.26
A3: 1B.9(C:I) B1.28
A4: 1C.2(A:I) B1.30
A5: 1C.12(D:I) B1.32
A6: 1C.5(B:I) B1.34
A7: 1C.9(C:I) B1.36
A8: 1D.2(A:I) B1.38
A9: 1D.12(D:I) B1.40
A10: 1D.5(B:I) B1.42
A11: 1D.9(C:I) B1.44
CHIPENABLE: 1E.2(A:I) B1.47
DUE_3.3: B1.3.3V J2.3 J2.4
DUE_5: J1.2 J2.5 J2.6
GND: 1B.1(A:OE) 1B.4(B:OE) 1B.10(C:OE) 1B.13(D:OE) 1C.1(A:OE) 1C.4(B:OE) 1C.10(C:OE) 1C.13(D:OE) 1D.1(A:OE) 1D.4(B:OE) 1D.10(C:OE) 1D.13(D:OE) 1E.1(A:OE) 1E.4(B:OE) 1E.10(C:OE) B1.GND@0(GND) B1.GND@1(GND) B1.GND@2(GND) B1.GND@3(GND) B1.GND@4(GND) D1.K(C) D2.K(C) D3.K(C) D4.K(C) D5.K(C) D6.K(C) J1.6 J2.1 J2.2 J2.15 J2.16 S1.1(S) S1.2(S1) ; supply symbol labelled SUP ; also sheet 1,2,3,4,6
I/O_0: B1.46 ; also sheet 2,3
I/O_1: B1.48 ; also sheet 2,3
I/O_2: B1.50 ; also sheet 2,3
I/O_3: B1.52 ; also sheet 2,3
LEDPIN: B1.13 R7.1
LSA0: 1B.3(A:O) ; also sheet 2,3
LSA1: 1B.11(D:O) ; also sheet 2,3
LSA2: 1B.6(B:O) ; also sheet 2,3
LSA3: 1B.8(C:O) ; also sheet 2,3
LSA4: 1C.3(A:O) ; also sheet 2,3
LSA5: 1C.11(D:O) ; also sheet 2,3
LSA6: 1C.6(B:O) ; also sheet 2,3
LSA7: 1C.8(C:O) ; also sheet 2,3
LSA8: 1D.3(A:O) ; also sheet 2,3
LSA9: 1D.11(D:O) ; also sheet 2,3
LSA10: 1D.6(B:O) ; also sheet 2,3
LSA11: 1D.8(C:O) ; also sheet 2,3
LSCHIPENABLE: 1E.3(A:O) ; also sheet 3
LSWHICHBUFFER: 1E.8(C:O) ; also sheet 2,3
LSWRITE: 1E.6(B:O) ; also sheet 3
N$24: D2.A R4.2
N$27: D4.A R6.2
N$28: D3.A R5.2
N$29: D1.A R3.2
N$34: D5.A R7.2
N$47: D6.A R8.2
RESET: B1.RESET S1.3(P) S1.4(P1)
RX: B1.0(0(RX0)) R6.1
RX2: B1.17(17(RX2)) ; also sheet 6
SD_CS: B1.53 J2.7 J2.8
SD_FAIL: B1.12 R8.1
SD_MISO: J1.1 J2.13 J2.14
SD_MOSI: J1.4 J2.9 J2.10
SD_SCK: J1.3 J2.11 J2.12
TX: B1.1(1(TX0)) R5.1
TX2: B1.16(16(TX2)) ; also sheet 6
VCC: R4.1 ; also sheet 2,3,6
WHICHBUFFER: 1E.9(C:I) B1.51
WRITE: 1E.5(B:I) B1.49
Unconnected: B1.2 B1.3 B1.4 B1.5 B1.5V@0(5V) B1.5V@1(5V) B1.5V@2(5V) B1.6 B1.7 B1.8 B1.9 B1.10 B1.11 B1.14(14(TX3)) B1.15(15(RX3)) B1.18(18(TX1)) B1.19(19(RX1)) B1.20(20(SDA)) B1.21(21(SCL)) B1.23 B1.25 B1.27 B1.29 B1.31 B1.33 B1.35 B1.37 B1.39 B1.41 B1.43 B1.45 B1.A0(A0(RX0)) B1.A1(A1(TX0)) B1.A2 B1.A3 B1.A4 B1.A5 B1.A6 B1.A7 B1.A8 B1.A9 B1.A10 B1.A11 B1.A12 B1.A13 B1.A14 B1.A15 B1.AREF J1.5

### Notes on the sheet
- Leds are 5mm, 2.2v 20ma green
  (I have an abundance of them)
- SD Card for DMD graphics
- DUE SPI header
- A

## Sheet 6 of 6: DMD Sync Control, Connectors
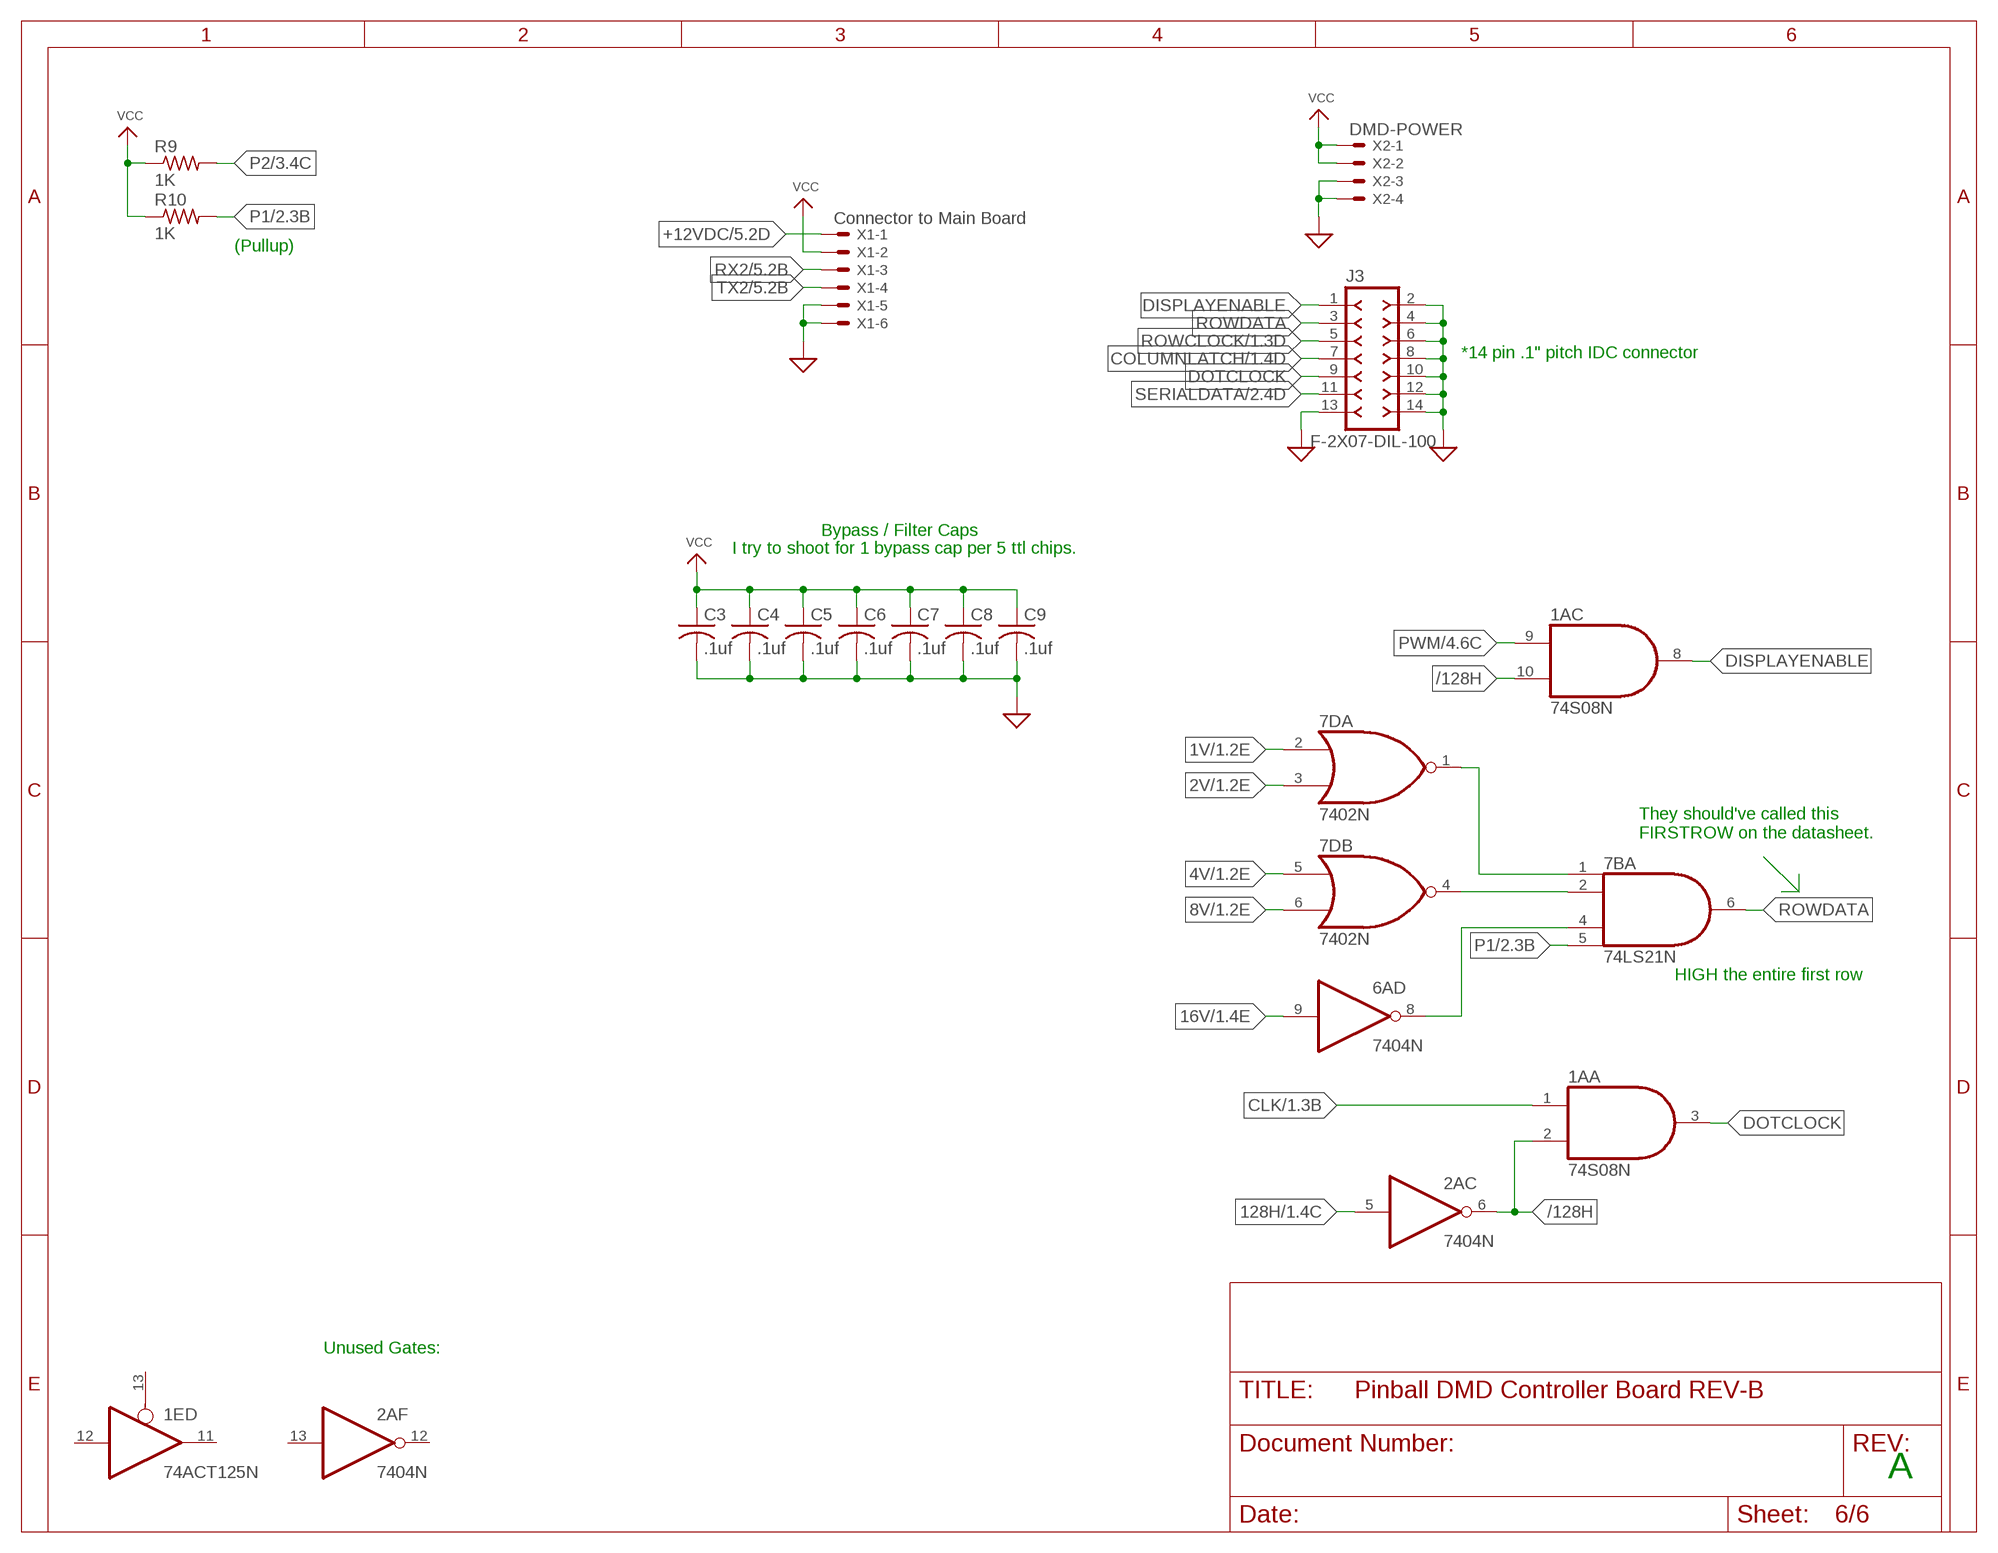
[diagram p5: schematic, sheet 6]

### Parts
C3  .1uf  C-US050-025X075  [C050-025X075]
C4  .1uf  C-US050-025X075  [C050-025X075]
C5  .1uf  C-US050-025X075  [C050-025X075]
C6  .1uf  C-US050-025X075  [C050-025X075]
C7  .1uf  C-US050-025X075  [C050-025X075]
C8  .1uf  C-US050-025X075  [C050-025X075]
C9  .1uf  C-US050-025X075  [C050-025X075]
J3  F-2X07-DIL-100  [DIL-100-2X07]
R9  1K  R-US_0204/7  [0204/7]
R10  1K  R-US_0204/7  [0204/7]
X1  Connector to Main Board  KK-156-6  [KK-156-6]
X2  DMD-POWER  KK-156-4  [KK-156-4]

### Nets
1V: 7D.2(A:I0) ; also sheet 1,2,3
2V: 7D.3(A:I1) ; also sheet 1,2,3
4V: 7D.5(B:I0) ; also sheet 1,2,3
8V: 7D.6(B:I1) ; also sheet 1,2,3
16V: 6A.9(D:I) ; also sheet 1,2,3
128H: 2A.5(C:I) ; also sheet 1
+12VDC: X1.1 ; also sheet 5
/128H: 1A.2(A:I1) 1A.10(C:I1) 2A.6(C:O)
CLK: 1A.1(A:I0) ; also sheet 1
COLUMNLATCH: J3.7 ; also sheet 1
DISPLAYENABLE: 1A.8(C:O) J3.1
DOTCLOCK: 1A.3(A:O) J3.9
GND: C3.2 C4.2 C5.2 C6.2 C7.2 C8.2 C9.2 J3.2 J3.4 J3.6 J3.8 J3.10 J3.12 J3.13 J3.14 X1.5 X1.6 X2.3 X2.4 ; supply symbol labelled SUP ; also sheet 1,2,3,4,5
N$11: 7B.1(A:I0) 7D.1(A:O)
N$12: 7B.2(A:I1) 7D.4(B:O)
N$13: 6A.8(D:O) 7B.4(A:I2)
P1: 7B.5(A:I3) R10.2 ; also sheet 2
P2: R9.2 ; also sheet 3
PWM: 1A.9(C:I0) ; also sheet 4
ROWCLOCK: J3.5 ; also sheet 1
ROWDATA: 7B.6(A:O) J3.3
RX2: X1.3 ; also sheet 5
SERIALDATA: J3.11 ; also sheet 2
TX2: X1.4 ; also sheet 5
VCC: C3.1 C4.1 C5.1 C6.1 C7.1 C8.1 C9.1 R9.1 R10.1 X1.2 X2.1 X2.2 ; also sheet 2,3,5
Unconnected: 1E.11(D:O) 1E.12(D:I) 1E.13(D:OE) 2A.12(F:O) 2A.13(F:I)

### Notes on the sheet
- (Pullup)
- *14 pin .1" pitch IDC connector
- Bypass / Filter Caps
- I try to shoot for 1 bypass cap per 5 ttl chips.
- They should've called this
  FIRSTROW on the datasheet.
- HIGH the entire first row
- Unused Gates:
- A

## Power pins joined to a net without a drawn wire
GND: 1A.7(P:GND) 1B.7(P:GND) 1C.7(P:GND) 1D.7(P:GND) 1E.7(P:GND) 2A.7(P:GND) 2B.10(GND) 2C.10(GND) 2D.10(GND) 2E.10(GND) 3A.8(GND) 3B.8(GND) 3C.8(GND) 3D.8(GND) 4A.10(GND) 4C.8(GND) 4D.8(GND) 4E.8(GND) 5A.8(GND) 5B.7(P:GND) 5C.8(GND) 5E.10(GND) 6A.7(P:GND) 6B.10(GND) 6C.8(GND) 6D.7(P:GND) 6E.7(P:GND) 7B.7(P:GND) 7C.7(P:GND) 7D.7(P:GND)
VCC: 1A.14(P:VCC) 1B.14(P:VCC) 1C.14(P:VCC) 1D.14(P:VCC) 1E.14(P:VCC) 2A.14(P:VCC) 2B.5(VCC) 2C.5(VCC) 2D.5(VCC) 2E.5(VCC) 3A.16(VCC) 3B.16(VCC) 3C.16(VCC) 3D.16(VCC) 4A.5(VCC) 4C.16(VCC) 4D.16(VCC) 4E.16(VCC) 5A.16(VCC) 5B.14(P:VCC) 5C.16(VCC) 5E.5(VCC) 6A.14(P:VCC) 6B.5(VCC) 6C.16(VCC) 6D.14(P:VCC) 6E.14(P:VCC) 7B.14(P:VCC) 7C.14(P:VCC) 7D.14(P:VCC)

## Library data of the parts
1A = 74xx-us:74*08: Quad 2-input AND gate
1B 1C 1D 1E 5B 6D = 74xx-us:74*125: Quad bus BUFFER, 3-state
2A 6A = 74xx-us:74*04: Hex INVERTER
2B 2C 2D 2E 4A 5E 6B = 74xx-us:74*93: Decade, divide by twelve and binary COUNTER
3A 3B 3C 3D 4C 4D 4E 5C = 74xx-us:74*157: Quadruple 2-line to 1-line data SELECTOR/MULTIPLEXER
4B 5D = OLD AND OBSOLETE ARCADE PARTS:7C168A-15PC: This is the 7C168A-15PC, a 4K x 4 CMOS RAM.
5A = 74xx-us:74*42: 4-line to 10-line DECODER (1-of-10)
6C = 74xx-us:74*153: Dual 4-line to 1-line data SELECTOR/MULTIPLEXER
6E = 74xx-us:74*11: Triple 3-input AND gate
7B = 74xx-us:74*21: Dual 4-input AND gate
7C = 74xx-us:74*107: Dual J-K FLIP FLOP, clear
7D = 74xx-us:74*02: Quad 2-input NOR gate
B1 = SparkFun-Boards:ARDUINO_MEGA_R3: Arduino Mega R3 ATmega2560 R3 compatible footprint. SparkFun Products: Arduino Mega 2560 R3
C1 C2 = BeagleBone_Black_Wireless:C-US: CAPACITOR, American symbol
C3-C9 = rcl:C-US: CAPACITOR, American symbol; SPICEPREFIX: C
D1-D6 = SparkFun-LED:LED: LED (Generic)
J1 = con-headers-jp:F-2X03-: FEMALE HEADER
J2 = con-headers-jp:F-2X08-: FEMALE HEADER
J3 = con-headers-jp:F-2X07-: FEMALE HEADER
Q1 = special:XTAL/S: CRYSTAL
R1 R2 R9 R10 = BeagleBone_Black_Wireless:R-US_: RESISTOR, American symbol
R3-R8 = rcl:R-US_: RESISTOR, American symbol; SPICEPREFIX: R
S1 = DC_LOAD_AU:10-XX: OMRON SWITCH; MPN: B3F-1000; OC_FARNELL: 176432; OC_NEWARK: 36M3542
X1 = con-molex:KK-156-6: KK 156 HEADER Source: http://www.molex.com/pdm_docs/sd/026604100_sd.pdf; MF: MOLEX; OC_FARNELL: unknown; OC_NEWARK: unknown
X2 = con-molex:KK-156-4: KK 156 HEADER Source: http://www.molex.com/pdm_docs/sd/026604100_sd.pdf; MF: MOLEX; OC_FARNELL: unknown; OC_NEWARK: unknown

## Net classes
0 default: width 0.406 mm, clearance 0.381 mm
